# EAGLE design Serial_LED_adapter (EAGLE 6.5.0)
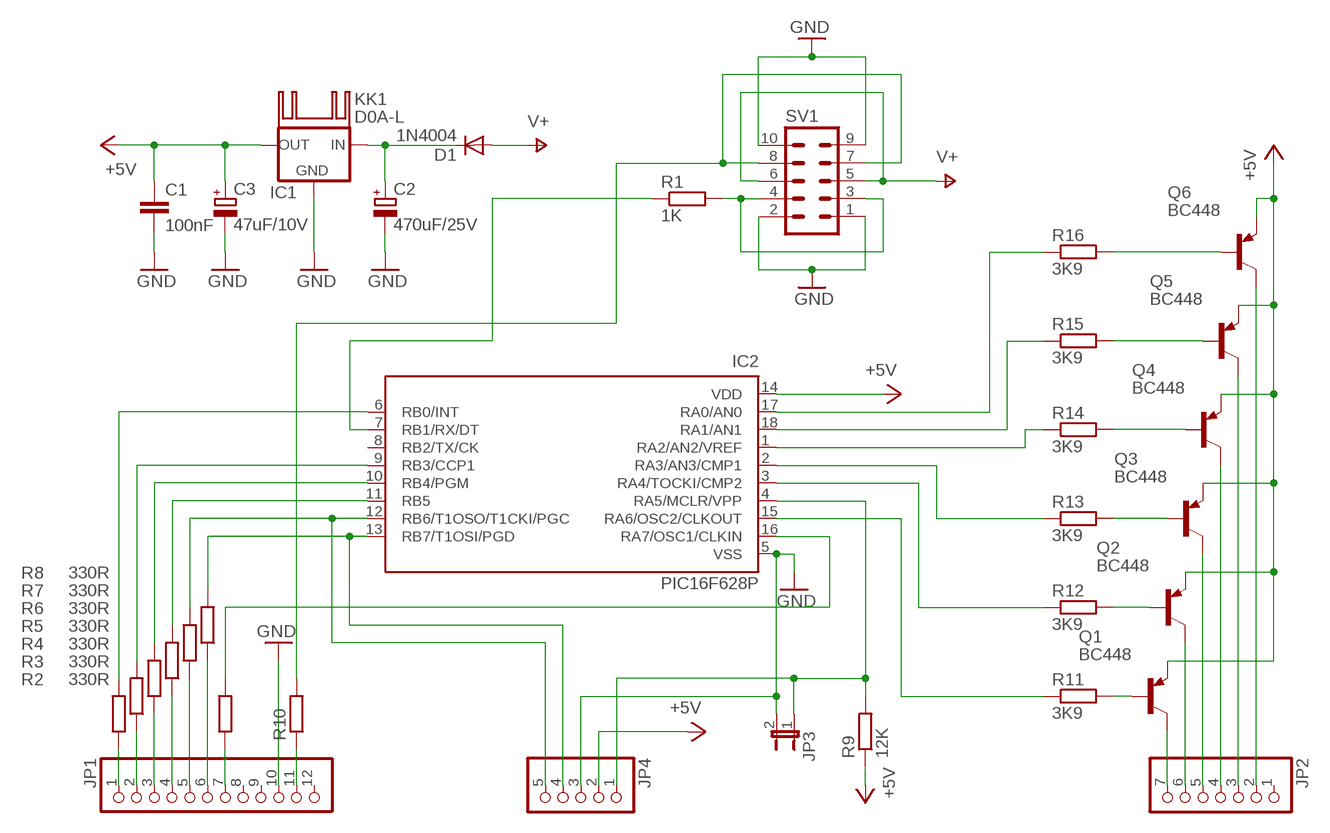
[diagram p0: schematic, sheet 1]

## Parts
C1  100nF  C-EUC025_050-024X070  [C025_050-024X070]
C2  470uF/25V  CPOL-EUE3.5-8  [E3,5-8]
C3  47uF/10V  CPOL-EUE2.5-5  [E2,5-5]
D1  1N4004  [DO41-10]
IC1  78XXL  [78XXL]
IC2  PIC16F628P  [DIL18]
JP1  PINHD-1X12  [1X12]
JP2  PINHD-1X7  [1X07]
JP3  JP1E  [JP1]
JP4  PINHD-1X5  [1X05]
KK1  D0A-L  [D02A-L]
Q1  BC448  [TO92-EBC]
Q2  BC448  [TO92-EBC]
Q3  BC448  [TO92-EBC]
Q4  BC448  [TO92-EBC]
Q5  BC448  [TO92-EBC]
Q6  BC448  [TO92-EBC]
R1  1K  R-EU_0207/10  [0207/10]
R2  330R  R-EU_0207/10  [0207/10]
R3  330R  R-EU_0207/10  [0207/10]
R4  330R  R-EU_0207/10  [0207/10]
R5  330R  R-EU_0207/10  [0207/10]
R6  330R  R-EU_0207/10  [0207/10]
R7  330R  R-EU_0207/10  [0207/10]
R8  330R  R-EU_0207/10  [0207/10]
R9  12K  R-EU_0207/10  [0207/10]
R10  R-EU_0207/10  [0207/10]
R11  3K9  R-EU_0207/10  [0207/10]
R12  3K9  R-EU_0207/10  [0207/10]
R13  3K9  R-EU_0207/10  [0207/10]
R14  3K9  R-EU_0207/10  [0207/10]
R15  3K9  R-EU_0207/10  [0207/10]
R16  3K9  R-EU_0207/10  [0207/10]
SV1  ML10  [ML10]

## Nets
+5V: C1.1 C3.+ IC1.OUT IC2.14(VDD) JP4.2 Q1.E Q2.E Q3.E Q4.E Q5.E Q6.E R9.1
GND: C1.2 C2.- C3.- IC1.GND IC2.5(VSS) JP1.10 JP3.2 JP4.3 SV1.1 SV1.2 SV1.9 SV1.10
N$1: IC2.15(RA6/OSC2/CLKOUT) R11.1
N$2: R10.2 SV1.7 SV1.8
N$3: IC2.3(RA4/TOCKI/CMP2) R12.1
N$4: IC2.2(RA3/AN3/CMP1) R13.1
N$5: R1.2 SV1.3 SV1.4
N$6: C2.+ D1.C IC1.IN
N$7: JP1.1 R2.1
N$8: JP1.2 R3.1
N$9: JP1.3 R4.1
N$10: JP1.4 R5.1
N$11: JP1.5 R6.1
N$12: JP1.6 R7.1
N$13: JP1.7 R8.1
N$14: IC2.6(RB0/INT) R2.2
N$15: IC2.9(RB3/CCP1) R3.2
N$16: IC2.10(RB4/PGM) R4.2
N$17: IC2.11(RB5) R5.2
N$18: IC2.12(RB6/T1OSO/T1CKI/PGC) JP4.5 R6.2
N$19: IC2.13(RB7/T1OSI/PGD) JP4.4 R7.2
N$20: IC2.16(RA7/OSC1/CLKIN) R8.2
N$21: IC2.7(RB1/RX/DT) R1.1
N$22: IC2.4(RA5/MCLR/VPP) JP3.1 JP4.1 R9.2
N$23: IC2.1(RA2/AN2/VREF) R14.1
N$24: JP1.11 R10.1
N$25: IC2.18(RA1/AN1) R15.1
N$26: JP2.7 Q1.C
N$27: JP2.6 Q2.C
N$28: JP2.5 Q3.C
N$29: JP2.4 Q4.C
N$30: JP2.3 Q5.C
N$31: JP2.2 Q6.C
N$32: IC2.17(RA0/AN0) R16.1
N$33: Q6.B R16.2
N$34: Q5.B R15.2
N$35: Q4.B R14.2
N$36: Q3.B R13.2
N$37: Q2.B R12.2
N$38: Q1.B R11.2
V+: D1.A SV1.5 SV1.6
Unconnected: IC2.8(RB2/TX/CK) JP1.8 JP1.9 JP1.12 JP2.1

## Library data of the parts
C1 = rcl:C-EU: CAPACITOR, European symbol
C2 C3 = rcl:CPOL-EU: POLARIZED CAPACITOR, European symbol
D1 = diode:1N4004: DIODE
IC1 = v-reg:78XXL: VOLTAGE REGULATOR
IC2 = microchip-6:PIC16F62*: FLASH-Based 8-Bit CMOS Microcontroller Source: http://ww1.microchip.com/downloads/en/DeviceDoc/40300C.pdf
JP1 = pinhead:PINHD-1X12: PIN HEADER
JP2 = pinhead:PINHD-1X7: PIN HEADER
JP3 = jumper:JP1E: JUMPER
JP4 = pinhead:PINHD-1X5: PIN HEADER
KK1 = heatsink:D0A-L: HEATSINK
Q1-Q6 = transistor-pnp:BC448*: PNP Transistror
R1-R16 = rcl:R-EU_: RESISTOR, European symbol
SV1 = con-harting-ml:ML10: HARTING; OC_FARNELL: unknown; OC_NEWARK: unknown

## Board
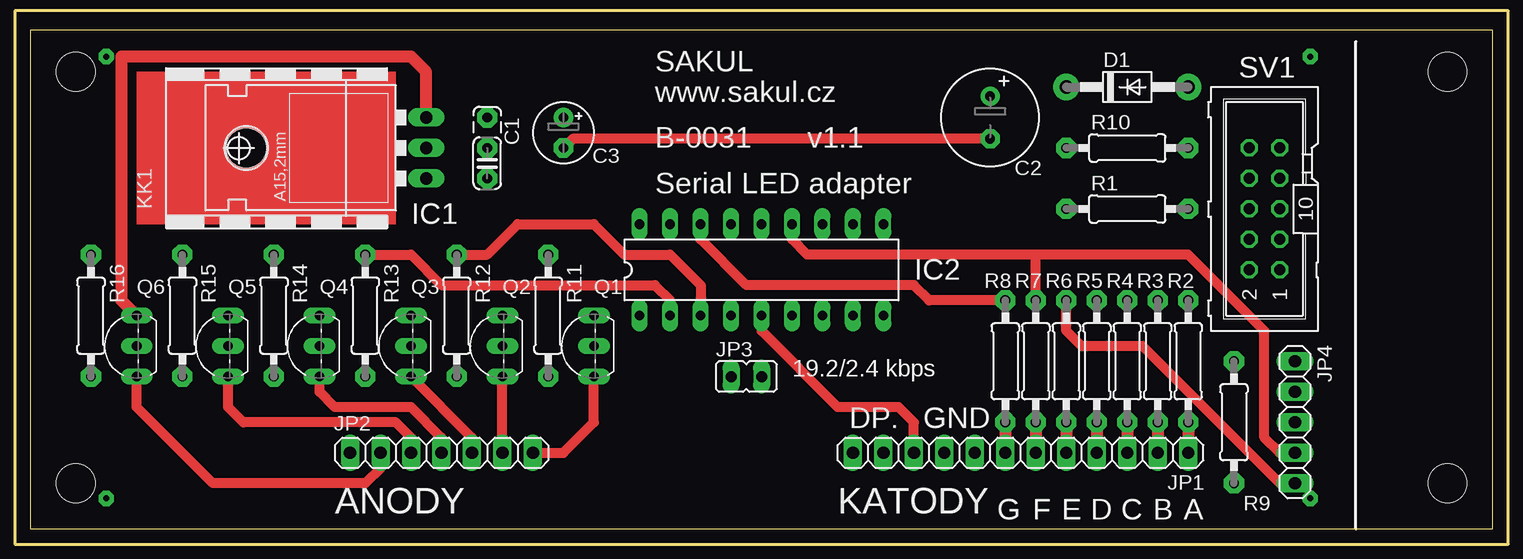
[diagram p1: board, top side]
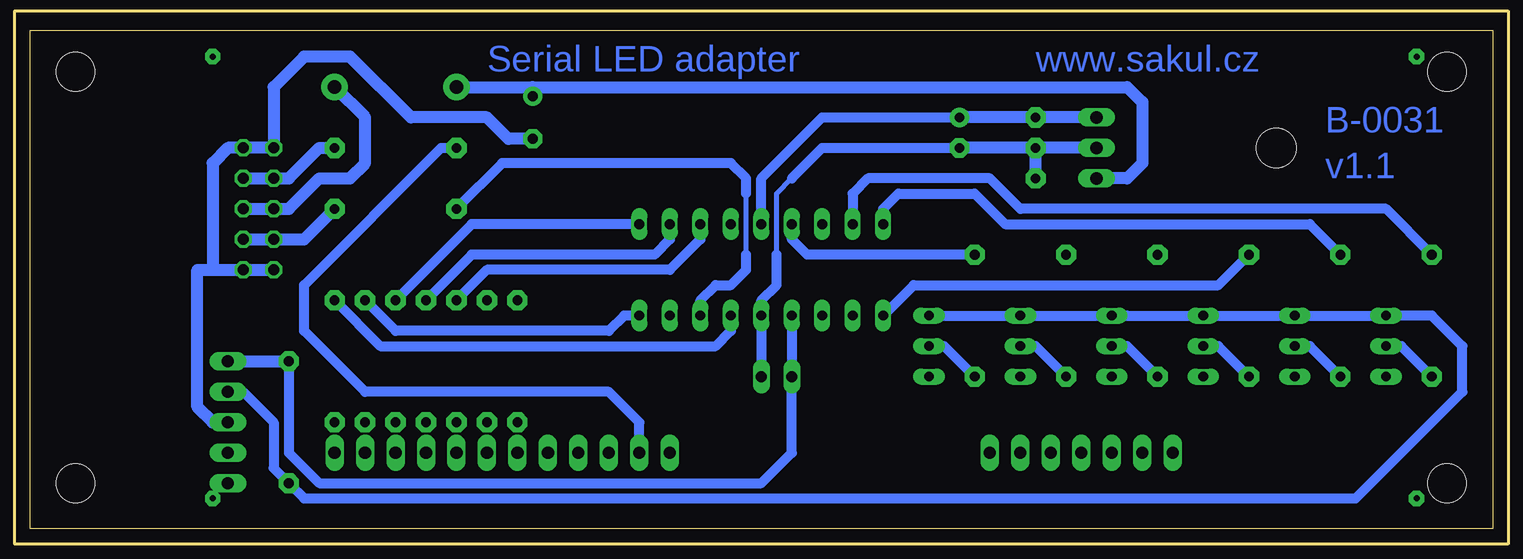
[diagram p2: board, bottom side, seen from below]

Size 121.9 x 41.58 mm. Coordinates in mm from the lower left corner, seen from the top.
Outline: 0,0 110.49,0 121.9,0 121.9,41.58 0,41.58 0,0
Copper layers (1*16): Top 0.035mm / dielectric 1.5mm / Bottom 0.035mm
Design rules "default": minimum track width 10mil, minimum drill 24mil, track to track 8mil, track to pad 8mil, pad to pad 8mil, via to via 8mil, smd to smd 8mil, copper to edge 40mil, drill to drill 8mil, minimum pad ring 10mil, minimum via ring 8mil, stop-mask expansion 4mil, vias tented up to drill 0mil, thermal gap 10mil
Holes 3.2 mm at 3.81,38.1 3.81,3.81 118.11,3.81 118.11,38.1
Milling: 4 lines

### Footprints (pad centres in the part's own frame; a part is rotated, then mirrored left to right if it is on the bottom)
C025_050-024X070 = drill 0.813 pad 1.676 octagon: 1 -3.81,0; 2 -1.27,0; 3 1.27,0
E3,5-8 = drill 0.813 pad 1.6: + -1.778,0 | drill 0.813 pad 1.6 octagon: - 1.778,0
E2,5-5 = drill 0.813 pad 1.6: + -1.27,0 | drill 0.813 pad 1.6 octagon: - 1.27,0
DO41-10 = drill 1.118 pad 2.184: A 5.08,0; C -5.08,0
78XXL = drill 1.016 long: GND 0,-3.81; IN -2.54,-3.81; OUT 2.54,-3.81 | hole 3.302: 0,11.176
DIL18 = drill 0.813 long: 1 -10.16,-3.81; 2 -7.62,-3.81; 3 -5.08,-3.81; 4 -2.54,-3.81; 5 0,-3.81; 6 2.54,-3.81; 7 5.08,-3.81; 8 7.62,-3.81; 9 10.16,-3.81; 10 10.16,3.81; 11 7.62,3.81; 12 5.08,3.81; 13 2.54,3.81; 14 0,3.81; 15 -2.54,3.81; 16 -5.08,3.81; 17 -7.62,3.81; 18 -10.16,3.81
1X12 = drill 1.016 long: 1 -13.97,0; 2 -11.43,0; 3 -8.89,0; 4 -6.35,0; 5 -3.81,0; 6 -1.27,0; 7 1.27,0; 8 3.81,0; 9 6.35,0; 10 8.89,0; 11 11.43,0; 12 13.97,0
1X07 = drill 1.016 long: 1 -7.62,0; 2 -5.08,0; 3 -2.54,0; 4 0,0; 5 2.54,0; 6 5.08,0; 7 7.62,0
JP1 = drill 0.914 long: 1 0,-1.27; 2 0,1.27
1X05 = drill 1.016 long: 1 -5.08,0; 2 -2.54,0; 3 0,0; 4 2.54,0; 5 5.08,0
TO92-EBC = drill 0.813 long: B 0,-1.27; C -2.54,-1.27; E 2.54,-1.27
0207/10 = drill 0.813 pad 1.676 octagon: 1 -5.08,0; 2 5.08,0
ML10 = drill 0.914 octagon: 1 -5.08,-1.27; 2 -5.08,1.27; 3 -2.54,-1.27; 4 -2.54,1.27; 5 0,-1.27; 6 0,1.27; 7 2.54,-1.27; 8 2.54,1.27; 9 5.08,-1.27; 10 5.08,1.27

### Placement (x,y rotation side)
C1  38.1,30.48 270 top
C2  80.01,34.29 270 top
C3  44.45,33.02 270 top
D1  91.44,36.83 0 top
IC1  29.21,31.75 90 top
IC2  60.96,21.59 0 top
JP1  82.55,6.35 180 top
JP2  34.29,6.35 0 top
JP3  59.69,12.7 270 top
JP4  105.41,8.89 270 top
KK1  22.86,31.75 0 top
Q1  45.72,15.24 90 top
Q2  38.1,15.24 90 top
Q3  30.48,15.24 90 top
Q4  22.86,15.24 90 top
Q5  15.24,15.24 90 top
Q6  7.62,15.24 90 top
R1  91.44,26.67 0 top
R2  96.52,13.97 90 top
R3  93.98,13.97 90 top
R4  91.44,13.97 90 top
R5  88.9,13.97 90 top
R6  86.36,13.97 90 top
R7  83.82,13.97 90 top
R8  81.28,13.97 90 top
R9  100.33,8.89 90 top
R10  91.44,31.75 0 top
R11  43.18,17.78 270 top
R12  35.56,17.78 270 top
R13  27.94,17.78 270 top
R14  20.32,17.78 270 top
R15  12.7,17.78 270 top
R16  5.08,17.78 270 top
SV1  102.87,26.67 90 top

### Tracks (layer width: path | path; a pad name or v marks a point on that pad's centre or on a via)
+5V
  Top 1.016: IC1.OUT 33.02,38.1 31.75,39.37 7.62,39.37 7.62,19.05 Q6.E
  Bottom 0.813: Q1.E Q2.E Q3.E | 30.48,17.78 Q3.E | Q3.E Q4.E Q5.E Q6.E 5.08,17.78 2.54,15.24 2.54,11.43 11.43,2.54 99.06,2.54 R9.1 101.6,5.08 101.6,8.89 104.14,11.43 JP4.2 | IC2.14 60.96,29.21 55.88,34.29 C3.+
  Bottom 1.016: IC1.OUT C1.1 C3.+
GND
  Top 0.813: JP1.10 73.66,8.89 72.39,10.16 67.31,10.16 60.96,16.51 IC2.5 | C2.- 45.21,32.51 C3.-
  Bottom 0.406: 59.69,22.86 59.69,27.94 58.42,29.21
  Bottom 0.813: JP3.2 IC2.5 60.96,19.05 59.69,20.32 59.69,22.86 | 58.42,29.21 55.88,31.75 C3.-
  Bottom 1.016: 106.68,21.59 106.68,30.48 105.41,31.75 SV1.9 SV1.10 101.6,36.83 99.06,39.37 95.25,39.37 90.17,34.29 83.82,34.29 82.04,32.51 C2.- | 106.68,21.59 SV1.1 SV1.2 | JP4.3 106.68,8.89 107.95,10.16 107.95,21.59 106.68,21.59 | IC1.GND C1.2 | 38.1,29.21 C1.2 | C1.2 C3.-
N$1
  Bottom 0.813: R11.1 57.15,22.86 58.42,24.13 IC2.15
N$2
  Bottom 1.016: SV1.7 SV1.8 100.33,29.21 97.79,31.75 R10.2
N$3
  Top 0.813: R12.1 38.1,22.86 40.64,25.4 46.99,25.4 49.53,22.86 53.34,22.86 55.88,20.32 IC2.3
N$4
  Top 0.813: R13.1 31.75,22.86 34.29,20.32 52.07,20.32 53.34,19.05 IC2.2
N$5
  Bottom 1.016: SV1.3 SV1.4 99.06,24.13 R1.2
N$6
  Bottom 1.016: D1.C 80.01,36.83 | 80.01,36.83 30.48,36.83 29.21,35.56 29.21,30.48 30.48,29.21 IC1.IN | C2.+ 80.01,36.83
N$7
  Top 1.016: R2.1 JP1.1
N$8
  Top 1.016: R3.1 JP1.2
N$9
  Top 1.016: R4.1 JP1.3
N$10
  Top 1.016: R5.1 JP1.4
N$11
  Top 1.016: R6.1 JP1.5
N$12
  Top 1.016: R7.1 JP1.6
N$13
  Top 1.016: R8.1 JP1.7
N$14
  Bottom 0.813: R2.2 92.71,15.24 64.77,15.24 63.5,16.51 IC2.6
N$15
  Bottom 0.813: IC2.9 72.39,17.78 73.66,16.51 91.44,16.51 R3.2
N$16
  Bottom 0.813: IC2.10 85.09,25.4 R4.2
N$17
  Bottom 0.813: IC2.11 68.58,24.13 69.85,22.86 85.09,22.86 R5.2
N$18
  Top 0.813: JP4.5 104.14,3.81 92.71,15.24 87.63,15.24 86.36,16.51 R6.2
  Bottom 0.813: IC2.12 66.04,24.13 68.58,21.59 83.82,21.59 R6.2
N$19
  Top 0.813: R7.2 83.82,22.86 | 83.82,22.86 64.77,22.86 63.5,24.13 IC2.13 | JP4.4 104.14,6.35 102.87,7.62 102.87,16.51 96.52,22.86 83.82,22.86
N$20
  Top 0.813: R8.2 74.93,19.05 73.66,20.32 59.69,20.32 55.88,24.13 IC2.16
N$21
  Bottom 0.406: 62.23,22.86 62.23,27.94
  Bottom 0.813: IC2.7 66.04,19.05 64.77,20.32 63.5,20.32 62.23,21.59 62.23,22.86 | 62.23,27.94 62.23,29.21 63.5,30.48 82.55,30.48 R1.1
N$22
  Bottom 0.813: IC2.4 JP3.1 58.42,6.35 60.96,3.81 97.79,3.81 100.33,6.35 R9.2
  Bottom 1.016: JP4.1 R9.2
N$23
  Bottom 0.813: IC2.1 48.26,20.32 22.86,20.32 R14.1
N$24
  Bottom 0.813: JP1.11 71.12,8.89 73.66,11.43 93.98,11.43 99.06,16.51 99.06,20.32 87.63,31.75 R10.1
N$25
  Bottom 0.813: IC2.18 50.8,26.67 49.53,27.94 43.18,27.94 40.64,25.4 15.24,25.4 R15.1
N$26
  Top 0.813: JP2.7 44.45,6.35 46.99,8.89 Q1.C
N$27
  Top 0.813: JP2.6 Q2.C
N$28
  Top 0.813: JP2.5 36.83,7.62 Q3.C
N$29
  Top 0.813: JP2.4 34.29,7.62 31.75,10.16 25.4,10.16 24.13,11.43 Q4.C
N$30
  Top 0.813: JP2.3 31.75,7.62 30.48,8.89 17.78,8.89 16.51,10.16 Q5.C
N$31
  Top 0.813: JP2.2 29.21,5.08 27.94,3.81 15.24,3.81 8.89,10.16 Q6.C
N$32
  Bottom 0.813: R16.1 8.89,26.67 39.37,26.67 41.91,29.21 52.07,29.21 53.34,27.94 IC2.17
N$33
  Bottom 0.813: Q6.B 7.62,15.24 R16.2
N$34
  Bottom 0.813: Q5.B 15.24,15.24 R15.2
N$35
  Bottom 0.813: Q4.B 22.86,15.24 R14.2
N$36
  Bottom 0.813: Q3.B 30.48,15.24 R13.2
N$37
  Bottom 0.813: Q2.B 38.1,15.24 R12.2
N$38
  Bottom 0.813: Q1.B 45.72,15.24 R11.2
N$39  (via drill 0.5 pad 1.27)
  other vias: 6.35,2.54
N$40  (via drill 0.5 pad 1.27)
  other vias: 6.35,39.37
N$41  (via drill 0.5 pad 1.27)
  other vias: 106.68,2.54
N$42  (via drill 0.5 pad 1.27)
  other vias: 106.68,39.37
V+
  Bottom 1.016: SV1.5 SV1.6 100.33,26.67 97.79,29.21 95.25,29.21 93.98,30.48 93.98,34.29 D1.A
(copper drawn outside any net)
  shapes: Top area x1

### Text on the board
Bottom: www.sakul.cz | Serial LED adapter | B-0031 | v1.1
tPlace: SAKUL | www.sakul.cz | B-0031 | v1.1 | Serial LED adapter | 19.2/2.4 kbps | DP. | GND | G | F | E | D | C | B | A | ANODY | KATODY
